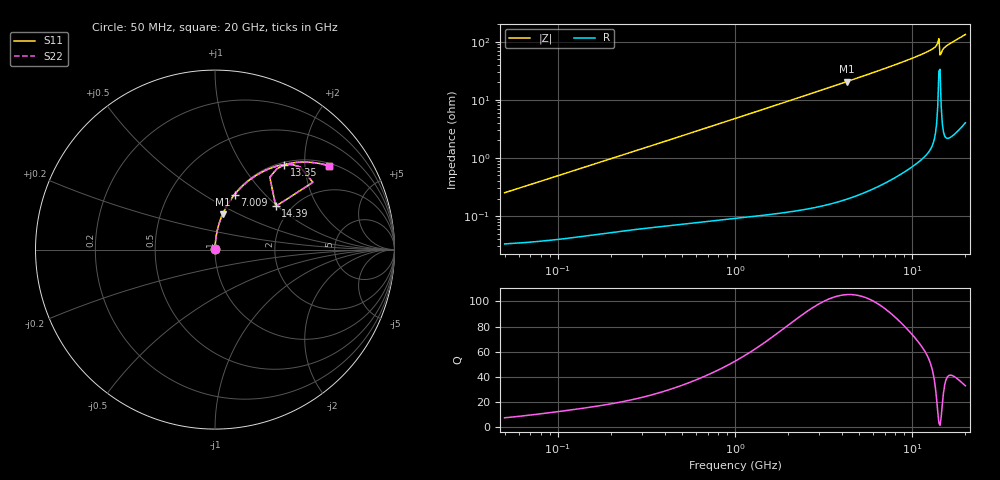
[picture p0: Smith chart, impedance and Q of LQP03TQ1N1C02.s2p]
!Murata Part Number: LQP03TQ1N1C02
!These Parameters are Measured in Series Mode Connection
!  o--[Z]--o
!Port1  Port2
!  o-------o
!Freq. Start=50[MHz] Stop=20[GHz], 401[Steps]
# Hz S RI R 50
!Freq.(Hz) S11(Real) S11(Imag) S21(Real) S21(Imag) S12(Real) S12(Imag) S22(Real) S22(Imag)
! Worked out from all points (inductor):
!   401 points, 50 MHz to 20 GHz, reference 50 ohm
!   read as one part in series: L = 790 pH near 51.52 MHz
!   highest Q = 105 at 4.276 GHz (marker M1), where L = 763 pH
!   S11 on the Smith chart (normalised r, x): 50 MHz: 1.00, +0.00; 7.009 GHz: 1.01, +0.69; 13.35 GHz: 1.04, +1.57; 14.39 GHz: 1.67, +0.97; 20 GHz: 1.08, +2.66
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5e7  0.000338 0.00249  0.9997 -0.00249  0.9997 -0.00249  0.000338 0.00249
1.364002e8  0.000489 0.00667  0.9995 -0.00667  0.9995 -0.00667  0.000489 0.00667
3.721004e8  0.00097 0.0178  0.999 -0.0178  0.999 -0.0178  0.00097 0.0178
1e9  0.00315 0.0473  0.9968 -0.0473  0.9968 -0.0473  0.00315 0.0473
1.714689e9  0.00765 0.0807  0.9923 -0.0807  0.9923 -0.0807  0.00765 0.0807
2.728004e9  0.0179 0.1273  0.9821 -0.1273  0.9821 -0.1273  0.0179 0.1273
4.275624e9  0.0421 0.1961  0.9579 -0.1961  0.9579 -0.1961  0.0421 0.1961
7.009217e9  0.1091 0.3065  0.8909 -0.3065  0.8909 -0.3065  0.1091 0.3065
7.442007e9  0.1223 0.3222  0.8777 -0.3222  0.8777 -0.3222  0.1223 0.3222
9.041845e9  0.1771 0.3756  0.8229 -0.3756  0.8229 -0.3756  0.1771 0.3756
1.066139e10  0.2416 0.4209  0.7584 -0.4209  0.7584 -0.4209  0.2416 0.4209
1.238412e10  0.3228 0.4585  0.6772 -0.4585  0.6772 -0.4585  0.3228 0.4585
1.334722e10  0.3853 0.4736  0.6147 -0.4736  0.6147 -0.4736  0.3853 0.4736
1.375312e10  0.4317 0.4736  0.5683 -0.4736  0.5683 -0.4736  0.4317 0.4736
1.396067e10  0.475 0.4605  0.525 -0.4605  0.525 -0.4605  0.475 0.4605
1.438523e10  0.3388 0.2413  0.6612 -0.2413  0.6612 -0.2413  0.3388 0.2413
1.460232e10  0.3052 0.4035  0.6948 -0.4035  0.6948 -0.4035  0.3052 0.4035
1.482269e10  0.3439 0.4488  0.6561 -0.4488  0.6561 -0.4488  0.3439 0.4488
1.504638e10  0.3714 0.4653  0.6286 -0.4653  0.6286 -0.4653  0.3714 0.4653
1.573793e10  0.4256 0.4819  0.5744 -0.4819  0.5744 -0.4819  0.4256 0.4819
1.747767e10  0.519 0.4873  0.481 -0.4873  0.481 -0.4873  0.519 0.4873
2e10  0.6346 0.4666  0.3654 -0.4666  0.3654 -0.4666  0.6346 0.4666
